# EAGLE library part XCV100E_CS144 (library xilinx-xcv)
xcv100e_cs144 edit this description Auto generated by make-symbol-device-package-bsdl.ulp Rev. 26 Source: xcv100e_cs144.bsd
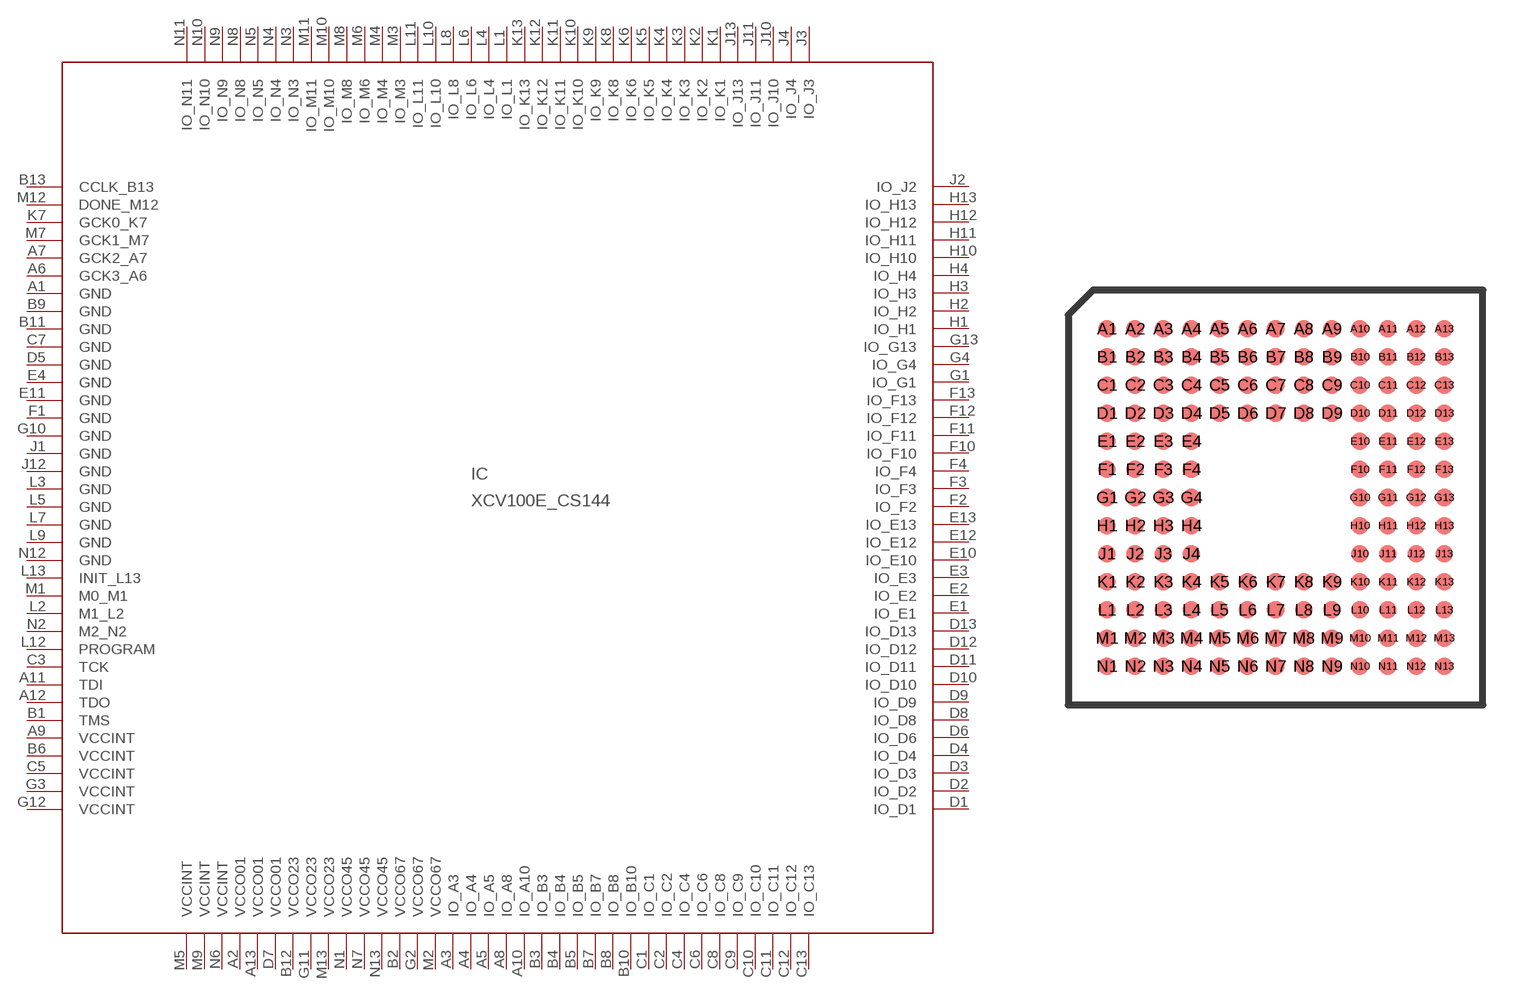
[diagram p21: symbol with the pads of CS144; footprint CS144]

Designator prefix IC

## XCV100E_CS144 (OC_FARNELL: unknown; OC_NEWARK: unknown)  [CS144]
A1  GND  pwr
A2  VCCO01  pwr
A3  IO_A3
A4  IO_A4
A5  IO_A5
A6  GCK3_A6  in
A7  GCK2_A7  in
A8  IO_A8
A9  VCCINT  pwr
A10  IO_A10
A11  TDI  in
A12  TDO  out
A13  VCCO01  pwr
B1  TMS  in
B2  VCCO67  pwr
B3  IO_B3
B4  IO_B4
B5  IO_B5
B6  VCCINT  pwr
B7  IO_B7
B8  IO_B8
B9  GND  pwr
B10  IO_B10
B11  GND  pwr
B12  VCCO23  pwr
B13  CCLK_B13
C1  IO_C1
C2  IO_C2
C3  TCK  in
C4  IO_C4
C5  VCCINT  pwr
C6  IO_C6
C7  GND  pwr
C8  IO_C8
C9  IO_C9
C10  IO_C10
C11  IO_C11
C12  IO_C12
C13  IO_C13
D1  IO_D1
D2  IO_D2
D3  IO_D3
D4  IO_D4
D5  GND  pwr
D6  IO_D6
D7  VCCO01  pwr
D8  IO_D8
D9  IO_D9
D10  IO_D10
D11  IO_D11
D12  IO_D12
D13  IO_D13
E1  IO_E1
E2  IO_E2
E3  IO_E3
E4  GND  pwr
E10  IO_E10
E11  GND  pwr
E12  IO_E12
E13  IO_E13
F1  GND  pwr
F2  IO_F2
F3  IO_F3
F4  IO_F4
F10  IO_F10
F11  IO_F11
F12  IO_F12
F13  IO_F13
G1  IO_G1
G2  VCCO67  pwr
G3  VCCINT  pwr
G4  IO_G4
G10  GND  pwr
G11  VCCO23  pwr
G12  VCCINT  pwr
G13  IO_G13
H1  IO_H1
H2  IO_H2
H3  IO_H3
H4  IO_H4
H10  IO_H10
H11  IO_H11
H12  IO_H12
H13  IO_H13
J1  GND  pwr
J2  IO_J2
J3  IO_J3
J4  IO_J4
J10  IO_J10
J11  IO_J11
J12  GND  pwr
J13  IO_J13
K1  IO_K1
K2  IO_K2
K3  IO_K3
K4  IO_K4
K5  IO_K5
K6  IO_K6
K7  GCK0_K7  in
K8  IO_K8
K9  IO_K9
K10  IO_K10
K11  IO_K11
K12  IO_K12
K13  IO_K13
L1  IO_L1
L2  M1_L2  in
L3  GND  pwr
L4  IO_L4
L5  GND  pwr
L6  IO_L6
L7  GND  pwr
L8  IO_L8
L9  GND  pwr
L10  IO_L10
L11  IO_L11
L12  PROGRAM  in
L13  INIT_L13
M1  M0_M1  in
M2  VCCO67  pwr
M3  IO_M3
M4  IO_M4
M5  VCCINT  pwr
M6  IO_M6
M7  GCK1_M7  in
M8  IO_M8
M9  VCCINT  pwr
M10  IO_M10
M11  IO_M11
M12  DONE_M12
M13  VCCO23  pwr
N1  VCCO45  pwr
N2  M2_N2  in
N3  IO_N3
N4  IO_N4
N5  IO_N5
N6  VCCINT  pwr
N7  VCCO45  pwr
N8  IO_N8
N9  IO_N9
N10  IO_N10
N11  IO_N11
N12  GND  pwr
N13  VCCO45  pwr

## Footprint CS144 (pad centres in mm)
xcv100e_cs144 edit this description Auto generated by make-symbol-device-package-bsdl.ulp Rev. 26 Source: xcv100e_cs144.bsd
smd 0.5 x 0.5: A1 -4.8,4.8; A2 -4,4.8; A3 -3.2,4.8; A4 -2.4,4.8; A5 -1.6,4.8; A6 -0.8,4.8; A7 0,4.8; A8 0.8,4.8; A9 1.6,4.8; A10 2.4,4.8; A11 3.2,4.8; A12 4,4.8; A13 4.8,4.8; B1 -4.8,4; B2 -4,4; B3 -3.2,4; B4 -2.4,4; B5 -1.6,4; B6 -0.8,4; B7 0,4; B8 0.8,4; B9 1.6,4; B10 2.4,4; B11 3.2,4; B12 4,4; B13 4.8,4; C1 -4.8,3.2; C2 -4,3.2; C3 -3.2,3.2; C4 -2.4,3.2; C5 -1.6,3.2; C6 -0.8,3.2; C7 0,3.2; C8 0.8,3.2; C9 1.6,3.2; C10 2.4,3.2; C11 3.2,3.2; C12 4,3.2; C13 4.8,3.2; D1 -4.8,2.4; D2 -4,2.4; D3 -3.2,2.4; D4 -2.4,2.4; D5 -1.6,2.4; D6 -0.8,2.4; D7 0,2.4; D8 0.8,2.4; D9 1.6,2.4; D10 2.4,2.4; D11 3.2,2.4; D12 4,2.4; D13 4.8,2.4; E1 -4.8,1.6; E2 -4,1.6; E3 -3.2,1.6; E4 -2.4,1.6; E10 2.4,1.6; E11 3.2,1.6; E12 4,1.6; E13 4.8,1.6; F1 -4.8,0.8; F2 -4,0.8; F3 -3.2,0.8; F4 -2.4,0.8; F10 2.4,0.8; F11 3.2,0.8; F12 4,0.8; F13 4.8,0.8; G1 -4.8,0; G2 -4,0; G3 -3.2,0; G4 -2.4,0; G10 2.4,0; G11 3.2,0; G12 4,0; G13 4.8,0; H1 -4.8,-0.8; H2 -4,-0.8; H3 -3.2,-0.8; H4 -2.4,-0.8; H10 2.4,-0.8; H11 3.2,-0.8; H12 4,-0.8; H13 4.8,-0.8; J1 -4.8,-1.6; J2 -4,-1.6; J3 -3.2,-1.6; J4 -2.4,-1.6; J10 2.4,-1.6; J11 3.2,-1.6; J12 4,-1.6; J13 4.8,-1.6; K1 -4.8,-2.4; K2 -4,-2.4; K3 -3.2,-2.4; K4 -2.4,-2.4; K5 -1.6,-2.4; K6 -0.8,-2.4; K7 0,-2.4; K8 0.8,-2.4; K9 1.6,-2.4; K10 2.4,-2.4; K11 3.2,-2.4; K12 4,-2.4; K13 4.8,-2.4; L1 -4.8,-3.2; L2 -4,-3.2; L3 -3.2,-3.2; L4 -2.4,-3.2; L5 -1.6,-3.2; L6 -0.8,-3.2; L7 0,-3.2; L8 0.8,-3.2; L9 1.6,-3.2; L10 2.4,-3.2; L11 3.2,-3.2; L12 4,-3.2; L13 4.8,-3.2; M1 -4.8,-4; M2 -4,-4; M3 -3.2,-4; M4 -2.4,-4; M5 -1.6,-4; M6 -0.8,-4; M7 0,-4; M8 0.8,-4; M9 1.6,-4; M10 2.4,-4; M11 3.2,-4; M12 4,-4; M13 4.8,-4; N1 -4.8,-4.8; N2 -4,-4.8; N3 -3.2,-4.8; N4 -2.4,-4.8; N5 -1.6,-4.8; N6 -0.8,-4.8; N7 0,-4.8; N8 0.8,-4.8; N9 1.6,-4.8; N10 2.4,-4.8; N11 3.2,-4.8; N12 4,-4.8; N13 4.8,-4.8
